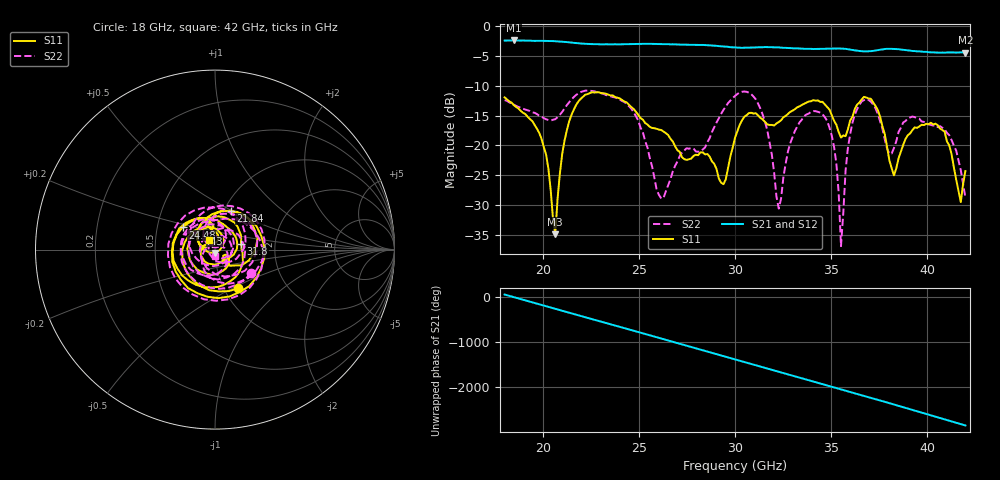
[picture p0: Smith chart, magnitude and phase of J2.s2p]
!Agilent Technologies,N5230A,US43500212,A.07.50.67
!Agilent N5230A: A.07.50.67
!Date: Monday, September 22, 2025 06:00:20
!Correction: S11(Full 2 Port(1,2))
!S21(Full 2 Port(1,2))
!S12(Full 2 Port(1,2))
!S22(Full 2 Port(1,2))
!S2P File: Measurements: S11, S21, S12, S22:
# Hz S  dB  R 50
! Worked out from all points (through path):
!   201 points, 18 GHz to 42 GHz, reference 50 ohm
!   highest |S21| = -2.43 dB at 18.48 GHz (marker M1); lowest = -4.5 dB at 42 GHz (marker M2)
!   lowest |S11| = -34.8 dB at 20.64 GHz (marker M3), VSWR 1.04, Z = 49.9 - j1.81 ohm
!   |S11| at or under -10 dB: start of sweep to end of sweep
!   |S22| runs from -36.8 to -10.8 dB; largest |S21 - S12| = 0.0067
!   S11 on the Smith chart (normalised r, x): 18 GHz: 1.17, -0.54; 21.84 GHz: 1.07, +0.49; 24.48 GHz: 0.68, +0.18; 31.8 GHz: 1.34, +0.08; 42 GHz: 0.93, +0.10
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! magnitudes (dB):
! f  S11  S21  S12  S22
! 18 GHz  -11.9  -2.4  -2.5  -12.4
! 18.48 GHz  -13.3  -2.4  -2.4  -13.2
! 19.92 GHz  -18.9  -2.5  -2.5  -15.2
! 20.64 GHz  -34.8  -2.6  -2.6  -15.6
! 21.12 GHz  -19.2  -2.7  -2.7  -13.8
! 21.84 GHz  -12.6  -2.9  -2.9  -11.3
! 22.08 GHz  -11.9  -3.0  -3.0  -10.9
! 24.48 GHz  -13.2  -3.1  -3.1  -13.4
! 26.04 GHz  -17.4  -3.0  -3.0  -28.3
! 29.4 GHz  -26.5  -3.4  -3.4  -14.0
! 30 GHz  -18.7  -3.6  -3.6  -11.7
! 31.8 GHz  -16.6  -3.5  -3.5  -19.5
! 32.28 GHz  -16.1  -3.6  -3.6  -30.6
! 34.08 GHz  -12.4  -3.9  -3.9  -14.3
! 35.16 GHz  -15.9  -3.8  -3.8  -20.2
! 35.52 GHz  -18.7  -3.8  -3.8  -36.8
! 35.88 GHz  -17.3  -3.9  -3.9  -20.4
! 36.36 GHz  -13.2  -4.1  -4.1  -13.9
! 38.04 GHz  -22.5  -3.8  -3.8  -21.4
! 40.68 GHz  -17.2  -4.5  -4.4  -16.8
! 41.76 GHz  -29.5  -4.4  -4.5  -24.1
! 42 GHz  -24.3  -4.5  -4.5  -28.7
